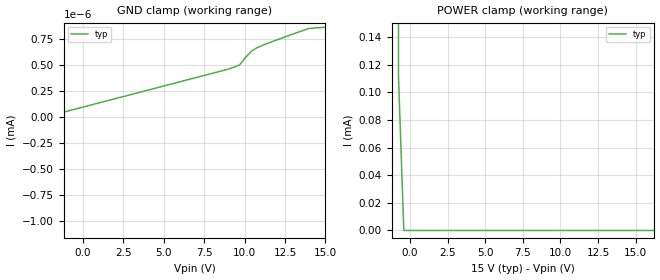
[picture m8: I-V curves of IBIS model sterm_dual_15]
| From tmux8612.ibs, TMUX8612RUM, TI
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| sterm_dual_15
[Model]   sterm_dual_15
Model_type   Terminator
|   typ   min   max
C_comp   6.362683e-12   NA   NA
[Voltage Range]   15   NA   NA
[Temperature Range]   27   NA   NA
[Power Clamp Reference]   15   NA   NA
[GND Clamp Reference]   0   NA   NA
[GND Clamp]
|   Voltage   I(typ)   I(min)   I(max)
-20V      -2.416A    NA         NA
-15.4V    -15.57nA   NA         NA
-15.05V   -514.1pA   NA         NA
8.99V     459.2pA    NA         NA
9.697V    500.3pA    NA         NA
10.4V     629.6pA    NA         NA
11.11V    687.7pA    NA         NA
13.94V    848.2pA    NA         NA
15V       860.8pA    NA         NA
[POWER Clamp]
|   Voltage   I(typ)   I(min)   I(max)
-5V       1.055A     NA         NA
-1.111V   25.67mA    NA         NA
-757.6mV  111.3uA    NA         NA
-404mV    1.903nA    NA         NA
30V       -512pA     NA         NA
